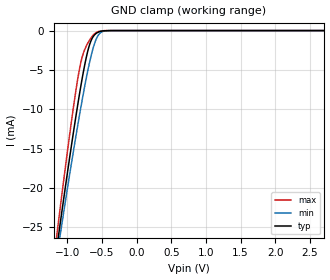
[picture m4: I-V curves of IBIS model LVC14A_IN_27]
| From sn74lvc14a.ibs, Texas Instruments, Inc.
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[Model]   LVC14A_IN_27
Model_type  Input
Vinh = 1.4
Vinl = 0.8
| variable   typ   min   max
C_comp   2.54pF   2.05pF   3.19pF
[Temperature Range]   40   100   -40
| Ambient temperature   25   85   -40
[Voltage range]   2.7   2.7   2.7
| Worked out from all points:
|   GND clamp passes 1 mA (typ) near -0.64 V on its own axis
[GND Clamp]
| LVC14A_IN_27
|   Voltage   I(typ)   I(min)   I(max)
-5.5V     -338.9mA   -314.3mA   -369mA
-1.165V   -28.41mA   -29.53mA   -26.91mA
-1.125V   -25.87mA   -27.21mA   -24.06mA
-1.09V    -23.67mA   -25.19mA   -21.6mA
-920mV    -13.36mA   -15.71mA   -10.21mA
-820mV    -7.797mA   -10.48mA   -4.654mA
-770mV    -5.293mA   -8.026mA   -2.891mA
-695mV    -2.253mA   -4.666mA   -1.432mA
-585mV    -362.1uA   -1.111mA   -263.9uA
-510mV    -78.77uA   -204.1uA   -38.82uA
-390mV    -3.679uA   -8.247uA   -639.4nA
2.7V      61.83pA    183.3pA    37.35pA
